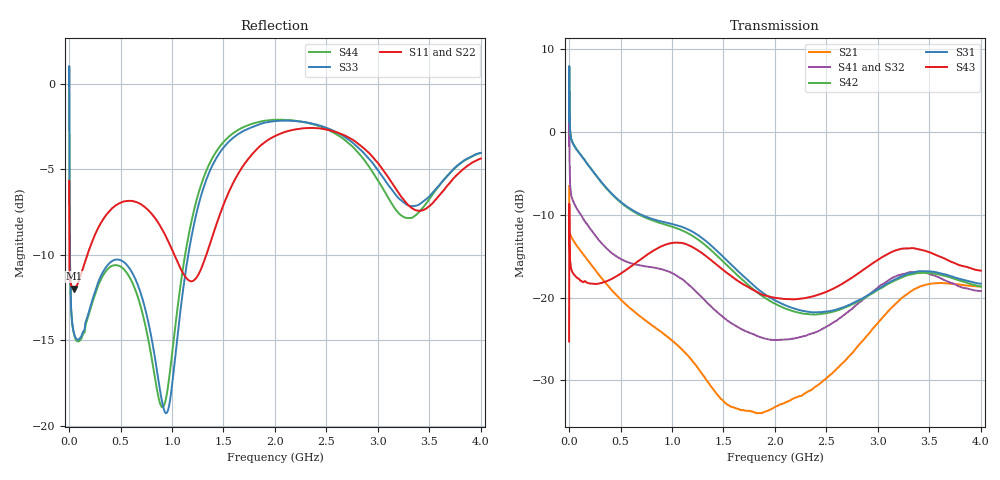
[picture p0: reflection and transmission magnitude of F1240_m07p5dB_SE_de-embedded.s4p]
! Integrated Device Technology
! Corporate Headquarters
! 6024 Silver Creek Valley Road
! San Jose, CA 95138  USA
! Phone:  1-408-284-8200
! Toll Free:  1-800-223-1366
! Webpage:  http://www.idt.com/
! Timing and RF Division
! 515 Groton Road, Suite 102
! Westford, MA 01886-6024
! Device:  F1240
! Description: Dual Intermediate Frequency Digital Variable Gain Amplifier
! Frequency:  10.0 -  500.00 MHz
! Package:  5x5 mm QFN Plastic Package: 32 pin
! Ports:  8 RF, 20 DC
!  Pin  1  = GA3 / Data  Pin 17  = RF OUT_B+
!  Pin  2  = GA4 / CLK  Pin 18  = RF OUT_B-
!  Pin  3  = GA5  Pin 19  = STBY_B
!  Pin  4  = VMODE  Pin 20  = Ground
!  Pin  5  = No Connect  Pin 21  = Ground
!  Pin  6  = GB5  Pin 22  = STB_A
!  Pin  7  = GB4  Pin 23  = RF OUT_A-  = Port 4
!  Pin  8  = GB3  Pin 24  = RF OUT_A+  = Port 3
!  Pin  9  = GB2  Pin 25  = GA0
!  Pin 10  = GB1  Pin 26  = ISET_A
!  Pin 11  = RF IN_B+  Pin 27  = VCC
!  Pin 12  = RF IN_B-  Pin 28  = Ground
!  Pin 13  = Ground  Pin 29  = RF IN_A-  = Port 2
!  Pin 14  = VCC  Pin 30  = RF IN_A+  = Port 1
!  Pin 15  = ISET_B  Pin 31  = GA1
!  Pin 16  = GB0  Pin 32  = GA2 / CSb
! Gain  = +19.5 dB
! State  = 1
! Voltage  = +5.00 V
! Current  = 85.292 mA (one channel only)
! Temperture  =  +25 C
! Test Date  =  2017-10-18
! Board  =  EB4031
! Data:  The device was measured on a custom evaluation board which has
!  individual transmission lines to the RF pins.  Data was collected
!  using a calibrated network analyzer.  The evaluation board was
!  de-embedded using Automatic Fixture Removal.
!  The reference plane is the edge of the package pin.
!  Only Channel A was measured.
!  This data is in single-ended operation.  If your needs are balanced
!  or differential S-parameters then this file needs to be used a
!  linear simulator.
! File Date:  2017-11-10  MJV
! Note:
!  Integrated Device Technology supplies this data as a sample of measured
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# Hz S dB R 100
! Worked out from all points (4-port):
!   410 points, 500 kHz to 4 GHz, reference 100 ohm
!   strongest paths, dB at 500 kHz, 930 MHz, 1.96 GHz, 2.98 GHz, 4 GHz:
!     S43: -25.3, -13.6, -19.9, -15.6, -16.8
!     S31: 1.2, -10.9, -20.1, -19.1, -18.3
!     S42: 1.2, -11.2, -20.5, -19.2, -18.7
!     S41: -1.7, -16.7, -25.1, -19.0, -19.2
!     S32: -1.7, -16.9, -24.9, -19.2, -19.5
!     S21: -6.5, -24.5, -33.5, -23.3, -18.7
!   lowest |S11| = -12.0 dB at 50 MHz (marker M1), VSWR 1.67, Z = 141 - j46.3 ohm
!   |S11| at or under -10 dB: 2.922 MHz to 178.1 MHz (175.1 MHz wide, 194 % of centre); 1.022 GHz to 1.334 GHz (311.5 MHz wide, 26.4 % of centre)
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500000  -5.68 -5.6  -6.54 -5.8  -31.55 77.8  -34.42 76.8
        -6.54 -5.8  -5.68 -5.6  -34.36 75.6  -31.56 78.9
        1.20 -110.7  -1.71 -112.7  -0.12 -0.0  -25.31 -39.0
        -1.73 -111.6  1.20 -109.5  -25.30 -39.2  -0.13 2.3
3500000  -10.51 -22.2  -11.62 -19.9  -24.29 5.3  -29.50 -10.7
         -11.63 -20.0  -10.50 -22.4  -29.47 -11.0  -24.29 5.5
         4.23 157.0  -1.01 140.9  -3.90 -82.7  -10.86 176.4
         -1.04 141.1  4.23 157.2  -10.87 176.4  -3.95 -82.6
5e7  -11.98 -37.6  -13.28 -22.9  -25.69 -17.3  -32.51 -20.4
     -13.28 -22.9  -11.93 -38.1  -32.52 -20.2  -25.65 -17.4
     -1.69 152.0  -8.67 142.6  -14.64 -163.7  -17.28 152.3
     -8.65 142.6  -1.63 151.8  -17.25 152.2  -14.71 -164.3
5e8  -6.96 -144.2  -20.21 -124.4  -29.29 -101.2  -36.91 -91.2
     -20.21 -124.3  -6.91 -145.1  -37.06 -89.1  -29.58 -101.1
     -8.42 29.6  -15.44 -18.5  -10.32 -173.2  -17.21 14.0
     -15.33 -19.9  -8.50 28.0  -17.12 13.7  -10.69 -173.9
2.06e9  -2.91 -179.8  -32.74 61.1  -33.06 -22.3  -35.25 -0.6
        -32.86 61.5  -2.81 179.8  -35.85 5.9  -34.54 -16.4
        -20.69 60.4  -25.00 -8.5  -2.17 175.0  -20.36 32.8
        -25.09 -15.8  -21.09 63.1  -20.13 33.9  -2.11 171.9
2.92e9  -4.09 100.4  -24.24 -27.8  -28.62 -156.7  -30.94 -142.5
        -24.24 -28.1  -3.88 101.2  -31.49 -129.2  -30.03 -148.8
        -19.57 -72.4  -19.83 -153.2  -4.44 92.5  -16.91 -93.4
        -19.57 -165.1  -19.66 -69.1  -16.11 -91.5  -4.91 85.0
4e9  -4.38 -127.3  -18.67 120.8  -27.36 -24.9  -28.38 -9.6
     -18.67 120.8  -4.13 -126.0  -28.94 4.0  -29.21 -14.7
     -18.32 52.0  -19.47 -42.8  -4.05 -133.1  -18.10 62.1
     -19.18 -57.2  -18.68 58.2  -16.75 55.6  -4.05 -143.0
